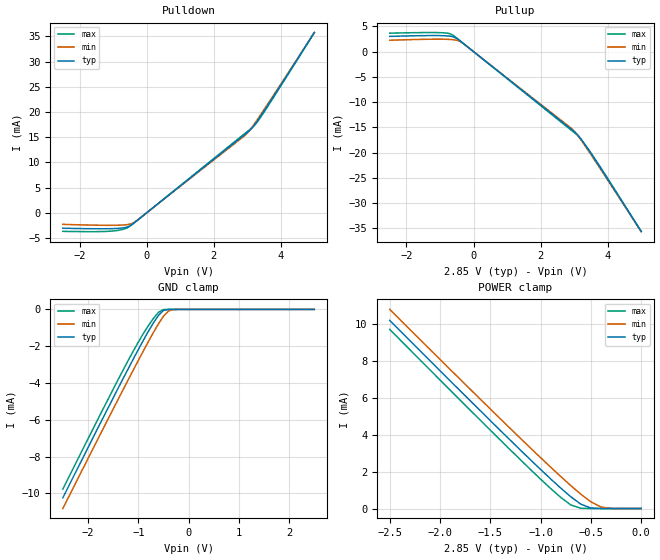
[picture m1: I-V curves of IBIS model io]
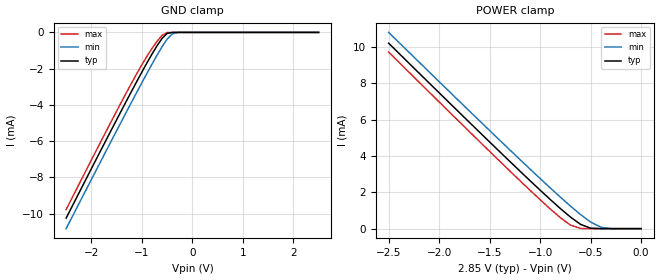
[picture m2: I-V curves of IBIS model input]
[IBIS Ver]	2.1
[File Name]	69r738c.ibs
[File Rev]	1.1
[Date]	8/31/99
[Source]	File originated at Motorola
[Notes]	This file is valid for:  MCM69R738C
|		(the 4M Late Write 2.5V I/O FSRAM).
[Disclaimer]This information is for modeling purposes only and
|		is not guaranteed.
[Component]		128Kx36FSRAM
[Manufacturer]	Motorola
[Package]
|  RLC Data is subject to change after further study of package
|		typ		min		max
R_pkg		100m		NA		NA
L_pkg		5nH		NA		NA
C_pkg		1.5pF		NA		NA
[Pin]		signal_name	model_name	R_pin		L_pin		C_pin
1A		VDDQ		POWER		NA		NA		NA
1B		NC		NC		NA		NA		NA
1C		NC		NC		NA		NA		NA
1D		DQc		io		NA		NA		NA
1E		DQc		io		NA		NA		NA
1F		VDDQ		POWER		NA		NA		NA
1G		DQc		io		NA		NA		NA
1H		DQc		io		NA		NA		NA
1J		VDDQ		POWER		NA		NA		NA
1K		DQd		io		NA		NA		NA
1L		DQd		io		NA		NA		NA
1M		VDDQ		POWER		NA		NA		NA
1N		DQd		io		NA		NA		NA
1P		DQd		io		NA		NA		NA
1R		NC		NC		NA		NA		NA
1T		NC		NC		NA		NA		NA
1U		VDDQ		POWER		NA		NA		NA
2A		SA		input		NA		NA		NA
2B		NC	 	NC		NA		NA		NA
2C		SA		input		NA		NA		NA
2D		DQc		io		NA		NA		NA
2E		DQc		io		NA		NA		NA
2F		DQc		io		NA		NA		NA
2G		DQc		io		NA		NA		NA
2H		DQc		io		NA		NA		NA
2J		VDD		POWER		NA		NA		NA
2K		DQd		io		NA		NA		NA
2L		DQd		io		NA		NA		NA
2M		DQd		io		NA		NA		NA
2N		DQd		io		NA		NA		NA
2P		DQd		io		NA		NA		NA
2R		SA		input		NA		NA		NA
2T		NC		NC		NA		NA		NA
2U		TMS		input		NA		NA		NA
3A		SA		input		NA		NA		NA
3B		SA		input		NA		NA		NA
3C		SA		input		NA		NA		NA
3D		VSS		GND		NA		NA		NA
3E		VSS		GND		NA		NA		NA
3F		VSS		GND		NA		NA		NA
3G		SBc#		input		NA		NA		NA
3H		VSS		GND		NA		NA		NA
3J		Vref		POWER		NA		NA		NA
3K		VSS		GND		NA		NA		NA
3L		SBd#		input		NA		NA		NA
3M		VSS		GND		NA		NA		NA
3N		VSS		GND		NA		NA		NA
3P		VSS		GND		NA		NA		NA
3R		VSS		GND		NA		NA		NA
3T		SA		input		NA		NA		NA
3U		TDI		input		NA		NA		NA
4A		NC		NC		NA		NA		NA
4B		NC		NC		NA		NA		NA
4C		VDD		POWER		NA		NA		NA
4D		ZQ		NC		NA		NA		NA
4E		SS#		input		NA		NA		NA
4F		G#		input		NA		NA		NA
4G		NC		NC		NA		NA		NA
4H		NC		NC		NA		NA		NA
4J		VDD		POWER		NA		NA		NA
4K		CK		input		NA		NA		NA
4L		CK#		input		NA		NA		NA
4M		SW#		input		NA		NA		NA
4N		SA		input		NA		NA		NA
4P		SA		input		NA		NA		NA
4R		VDD		POWER		NA		NA		NA
4T		SA		input		NA		NA		NA
4U		TCK		input		NA		NA		NA
5A		SA		input		NA		NA		NA
5B		SA		input		NA		NA		NA
5C		SA		input		NA		NA		NA
5D		VSS		GND		NA		NA		NA
5E		VSS		GND		NA		NA		NA
5F		VSS		GND		NA		NA		NA
5G		SBb#		input		NA		NA		NA
5H		VSS		GND		NA		NA		NA
5J		Vref		POWER		NA		NA		NA
5K		VSS		GND		NA		NA		NA
5L		SBa#		input		NA		NA		NA
5M		VSS		GND		NA		NA		NA
5N		VSS		GND		NA		NA		NA
5P		VSS		GND		NA		NA		NA
5R		VDD		POWER		NA		NA		NA
5T		SA		input		NA		NA		NA
5U		TDO		input		NA		NA		NA
6A		SA		input		NA		NA		NA
6B		NC		NC		NA		NA		NA
6C		SA		input		NA		NA		NA
6D		DQb		io		NA		NA		NA
6E		DQb		io		NA		NA		NA
6F		DQb		io		NA		NA		NA
6G		DQb		io		NA		NA		NA
6H		DQb		io		NA		NA		NA
6J		VDD		POWER		NA		NA		NA
6K		DQa		io		NA		NA		NA
6L		DQa		io		NA		NA		NA
6M		DQa		io		NA		NA		NA
6N		DQa		io		NA		NA		NA
6P		DQa		io		NA		NA		NA
6R		SA		input		NA		NA		NA
6T		NC		NC		NA		NA		NA
6U		NC		NC		NA		NA		NA
7A		VDDQ		POWER		NA		NA		NA
7B		NC		NC		NA		NA		NA
7C		NC		NC		NA		NA		NA
7D		DQb		io		NA		NA		NA
7E		DQb		io		NA		NA		NA
7F		VDDQ		POWER		NA		NA		NA
7G		DQb		io		NA		NA		NA
7H		DQb		io		NA		NA		NA
7J		VDDQ		POWER		NA		NA		NA
7K		DQa		io		NA		NA		NA
7L		DQa		io		NA		NA		NA
7M		VDDQ		POWER		NA		NA		NA
7N		DQa		io		NA		NA		NA
7P		DQa		io		NA		NA		NA
7R		NC		NC		NA		NA		NA
7T		NC		NC		NA		NA		NA
7U		VDDQ		POWER		NA		NA		NA
| Models and submodels in the file (2): io (I/O), input (Input)
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[Model]	io
Model_type	I/O
Polarity	Non-Inverting
Enable	Active-Low
|		signals  DQa, DQb, DQc, DQd
|		typ		min		max
C_comp	6pF		5pF		8pF
|   |   |\ |   Rref
|   |Driver| \|------o----/\/\/\----o Vref
|   |   | /|   |
|   |   |/ |   === Cref
|   GND
Cref = 20pF
Rref = 50
Vref = 1.25
Vmeas = 1.25
Vinl = 0.65
Vinh = 1.75
|			typ		min		max
[Voltage range]	2.85V		2.7V		3.0V
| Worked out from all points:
|   slope of the pulldown table from 0 to 0.427 V, typ, clamps not added: 188 ohm
|   slope of the pullup table from 0 to 0.427 V, typ, clamps not added: 189 ohm
|   GND clamp passes 1 mA (typ) near -0.76 V on its own axis
|   POWER clamp passes 1 mA (typ) near -0.78 V on its own axis
| Temperature   50 C		110 C		0 C
[Pullup]
|	Voltage  	I(typ)   I(min)   I(max)
-2.5V     3.02mA     2.252mA    3.658mA
-800mV    3.126mA    2.442mA    3.678mA
-600mV    2.94mA     2.357mA    3.201mA
-400mV    2.117mA    2.008mA    2.142mA
-300mV    1.588mA    1.562mA    1.606mA
3V        -15.84mA   -15.72mA   -16.02mA
3.2V      -17.27mA   -17.44mA   -17.33mA
3.5V      -20.15mA   -20.38mA   -20.07mA
4V        -25.25mA   -25.43mA   -25.13mA
5V        -35.62mA   -35.67mA   -35.61mA
[Pulldown]
|	Voltage  	I(typ)   I(min)   I(max)
-2.5V     -3.055mA   -2.289mA   -3.68mA
-1.4V     -3.17mA    -2.466mA   -3.724mA
-900mV    -3.109mA   -2.468mA   -3.53mA
-600mV    -2.864mA   -2.363mA   -3.07mA
-400mV    -2.127mA   -2.013mA   -2.154mA
-300mV    -1.598mA   -1.569mA   -1.615mA
3V        15.93mA    15.79mA    16.12mA
3.2V      17.27mA    17.5mA     17.22mA
3.4V      19.18mA    19.45mA    18.96mA
5V        35.74mA    35.75mA    35.73mA
|   TRI-STATED OUTPUT
|   typ		min		max
|Voltage range	2.85V		2.7V		3.0V
| Temperature   50 C		110 C		0 C
|****************  FOR OUTPUTS  *********
[GND_clamp]
|	Voltage  	I(typ)   I(min)   I(max)
-2.5V     -10.24mA   -10.82mA   -9.77mA
-1.5V     -4.816mA   -5.419mA   -4.341mA
-1.2V     -3.223mA   -3.823mA   -2.771mA
-1V       -2.186mA   -2.776mA   -1.779mA
-800mV    -1.195mA   -1.753mA   -885uA
-600mV    -331.4uA   -790uA     -160.2uA
-500mV    -55.12uA   -375.1uA   -9.724uA
-400mV    -3.42uA    -89.37uA   -353.7nA
-300mV    -172.7nA   -7.306uA   -11.64nA
-200mV    -8.594nA   -415.9nA   -359pA
2.5V      29.74pA    1.668nA    2.913pA
[POWER_clamp]
|	Voltage  	I(typ)   I(min)   I(max)
-2.5V     10.22mA    10.81mA    9.729mA
-1.2V     3.171mA    3.809mA    2.645mA
-900mV    1.609mA    2.246mA    1.087mA
-800mV    1.11mA     1.739mA    605.8uA
-700mV    639.4uA    1.246mA    195.9uA
-600mV    237uA      778.6uA    11.41uA
-500mV    25.6uA     364uA      177.5nA
-400mV    828.2nA    82.27uA    2.542nA
-300mV    22.98nA    6.041uA    39.81pA
0V        29.74pA    1.668nA    2.913pA
[Ramp]
| 		typ			min			max
|Temperature  50 C		110 C			0 C
dV/dt_r	0.313/0.245n	0.309/0.257n	0.316/0.232n
dV/dt_f	0.312/0.193n	0.311/0.236n	0.318/0.117n
[Model]		input
Model_type		Input
Polarity		Non-Inverting
| signals  SA, G#,  SS#, SBa#, SBb#, SBc#, SBd#, CK#, CK,
|   TDI,  TMS,  TCK, SW#, ZQ, TDO
|  	* TDO has been listed here, but it is technically an output pin.
| 	This simplification has been made under the assumption
|  	that its structure is similar to the input pin's structure.
Vinl = 0.65V
Vinh = 1.75V
|			typ		min		max
C_comp		5pF		4pF		5pF
|			typ		min		max
[Voltage range]	2.85V		2.70V		3.0V
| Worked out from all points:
|   GND clamp passes 1 mA (typ) near -0.76 V on its own axis
|   POWER clamp passes 1 mA (typ) near -0.78 V on its own axis
| Temperature   50 C		110 C		0 C
[GND_clamp]
|	Voltage  	I(typ)   I(min)   I(max)
-2.5V     -10.24mA   -10.82mA   -9.77mA
-1.5V     -4.816mA   -5.419mA   -4.341mA
-1.2V     -3.223mA   -3.823mA   -2.771mA
-1V       -2.186mA   -2.776mA   -1.779mA
-800mV    -1.195mA   -1.753mA   -885uA
-600mV    -331.4uA   -790uA     -160.2uA
-500mV    -55.12uA   -375.1uA   -9.724uA
-400mV    -3.42uA    -89.37uA   -353.7nA
-300mV    -172.7nA   -7.306uA   -11.64nA
-200mV    -8.594nA   -415.9nA   -359pA
2.5V      29.74pA    1.668nA    2.913pA
[POWER_clamp]
|	Voltage  	I(typ)   I(min)   I(max)
-2.5V     10.22mA    10.81mA    9.729mA
-1.2V     3.171mA    3.809mA    2.645mA
-900mV    1.609mA    2.246mA    1.087mA
-800mV    1.11mA     1.739mA    605.8uA
-700mV    639.4uA    1.246mA    195.9uA
-600mV    237uA      778.6uA    11.41uA
-500mV    25.6uA     364uA      177.5nA
-400mV    828.2nA    82.27uA    2.542nA
-300mV    22.98nA    6.041uA    39.81pA
0V        29.74pA    1.668nA    2.913pA
